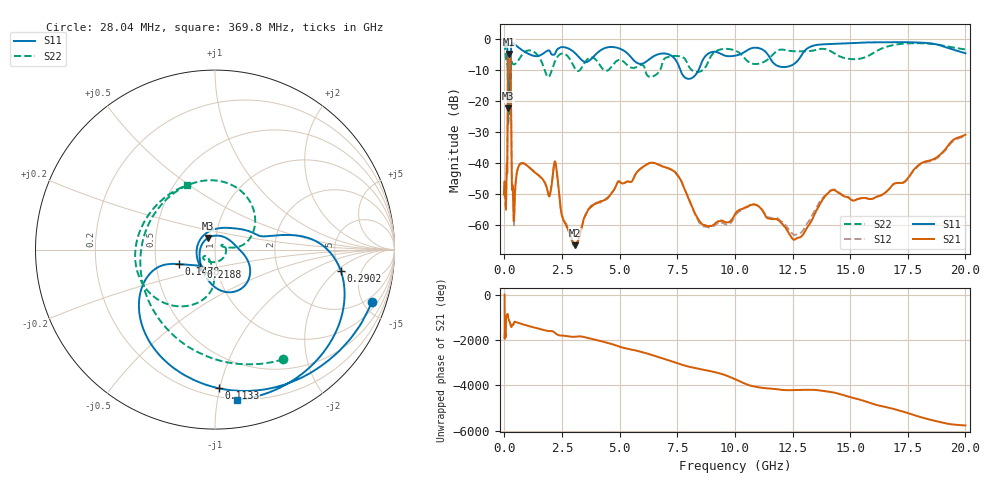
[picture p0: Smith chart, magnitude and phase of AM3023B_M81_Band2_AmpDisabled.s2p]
!Agilent Technologies,E8364B,MY43040894,A.07.50.67
!Agilent E8364B: A.07.50.67
!Date: Tuesday, October 27, 2020 10:39:21
!Correction: S11(Full 2 Port(1,2))
!S21(Full 2 Port(1,2))
!S12(Full 2 Port(1,2))
!S22(Full 2 Port(1,2))
!S2P File: Measurements: S11, S21, S12, S22:Log Frequency Sweep
# Hz S  dB  R 50
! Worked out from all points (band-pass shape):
!   3201 points, 10 MHz to 20 GHz, reference 50 ohm
!   highest |S21| = -4.88 dB at 191.5 MHz (marker M1); lowest = -66.7 dB at 3.07 GHz (marker M2)
!   |S21| within 3 dB of the highest: 152.9 MHz to 264.8 MHz (111.9 MHz wide, 53.6 % of centre)
!   lowest |S11| = -22.4 dB at 173.3 MHz (marker M3), VSWR 1.16, Z = 46 + j6.04 ohm
!   |S11| at or under -10 dB: 144.7 MHz to 262.5 MHz (117.8 MHz wide, 57.9 % of centre); 7.627 GHz to 8.431 GHz (804.1 MHz wide, 10 % of centre)
!   |S22| runs from -27.7 to -1.3 dB; largest |S21 - S12| = 0.009
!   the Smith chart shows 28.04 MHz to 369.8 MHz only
!   S11 on the Smith chart (normalised r, x): 28.04 MHz: 1.49, -5.76; 113.3 MHz: 0.26, -0.99; 147.8 MHz: 0.66, -0.11; 218.8 MHz: 0.83, -0.17; 290.2 MHz: 4.78, -2.27; 369.8 MHz: 0.19, -1.14
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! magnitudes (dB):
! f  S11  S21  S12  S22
! 10 MHz  -0.6  -47.7  -47.5  -1.3
! 28.04 MHz  -0.7  -48.9  -48.7  -2.9
! 35.55 MHz  -0.8  -49.4  -48.6  -3.6
! 68.48 MHz  -1.1  -54.5  -54.4  -6.3
! 113.3 MHz  -2.2  -40.6  -40.6  -8.1
! 126.1 MHz  -3.1  -40.9  -41.1  -8.2
! 147.8 MHz  -13.3  -11.1  -11.2  -11.2
! 173.3 MHz  -22.4  -5.3  -5.3  -25.3
! 191.5 MHz  -12.9  -4.9  -4.9  -23.5
! 218.8 MHz  -17.9  -5.2  -5.2  -22.0
! 290.2 MHz  -3.0  -21.6  -21.6  -7.0
! 324.5 MHz  -1.5  -46.6  -46.2  -7.6
! 369.8 MHz  -1.4  -49.0  -48.7  -8.1
! 409.6 MHz  -1.6  -58.7  -60.1  -8.3
! 447.2 MHz  -1.8  -51.8  -52.0  -8.2
! 672.9 MHz  -3.2  -40.4  -40.7  -6.2
! 1.59 GHz  -5.2  -44.7  -44.9  -7.0
! 2.212 GHz  -4.7  -39.9  -39.8  -7.0
! 3.07 GHz  -4.7  -66.7  -66.4  -9.7
! 5.639 GHz  -7.1  -44.4  -44.5  -9.4
! 12.71 GHz  -7.2  -64.2  -63.0  -4.1
! 20 GHz  -4.7  -30.9  -31.3  -3.5
